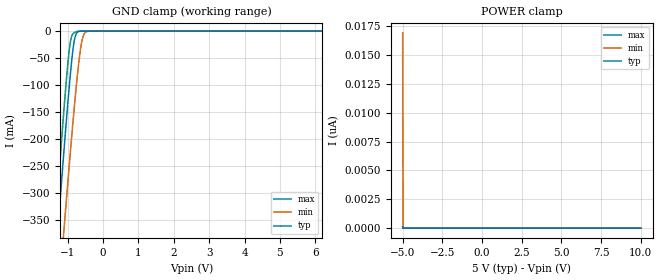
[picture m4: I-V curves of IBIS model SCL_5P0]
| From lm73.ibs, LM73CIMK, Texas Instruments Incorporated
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|   Model SCL_5P0
[Model]   SCL_5P0
Model_type   Input
Vinl = 1.5
Vinh = 3.5
|   typ   min   max
|   (nom PVT)   (fast PVT)   (slow PVT)
C_comp   0.4295pF   0.3981pF   0.4645pF
[Model spec]
|subparameter
Vinl   1.5   1.35   1.65
Vinh   3.5   3.15   3.85
[Voltage Range]   5   4.5   5.5
[Temperature Range]   27   150   -40
[Power Clamp Reference]   5   4.5   5.5
[GND Clamp Reference]   0   0   0
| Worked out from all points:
|   GND clamp passes 1 mA (typ) near -0.69 V on its own axis
[GND Clamp]
|   Voltage   I(typ)   I(min)   I(max)
-5V       -3.717A    -3.696A    -3.741A
-1.355V   -440.5mA   -580.4mA   -367.5mA
-1.25V    -349mA     -492.5mA   -273.8mA
-1.1V     -221.4mA   -368.7mA   -144.7mA
-995mV    -136.3mA   -284mA     -63.12mA
-920mV    -80.35mA   -225mA     -20.38mA
-830mV    -26.44mA   -157mA     -4.067mA
-755mV    -5.133mA   -104mA     -1.322mA
-665mV    -541.8uA   -49.06mA   -194.9uA
-590mV    -80.07uA   -17.34mA   -24.67uA
-425mV    -675.3nA   -383.9uA   -57.47nA
10V       0A         0A         0A
[POWER Clamp]
|   Voltage   I(typ)   I(min)   I(max)
-5V       125.3pA    16.91nA    115.7pA
-4.97V    0A         0A         0A
-4.955V   0A         0A         0A
10V       0A         0A         0A
